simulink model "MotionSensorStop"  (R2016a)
settings: Solver=VariableStepAuto  StartTime=0.0  StopTime=10.0  RelTol=1e-3
libraries: vexarmcortexlib x3

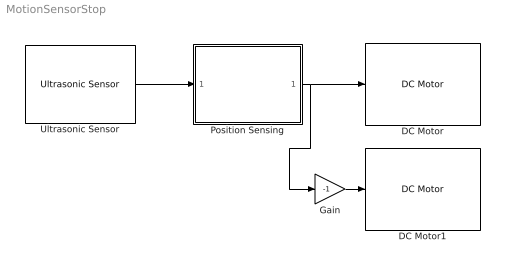
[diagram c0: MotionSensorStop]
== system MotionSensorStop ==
  DC Motor : vexarmcortexlib/DC Motor  motor=3  scaleFactor=1/13.5  SimulationOut=off
  DC Motor1 : vexarmcortexlib/DC Motor  motor=7  scaleFactor=1/13.5  SimulationOut=off
  Gain : Gain  Gain=-1
  Position Sensing : Stateflow chart  TreatAsAtomicUnit=on
  Ultrasonic Sensor : vexarmcortexlib/Ultrasonic Sensor  inputPin=3  outputPin=2  inputPortSim=off  SampleTime=0.2
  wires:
  Ultrasonic Sensor/1 -> Position Sensing/1(position)
  Position Sensing/1(speed) -> Gain/1, DC Motor/1
  Gain/1 -> DC Motor1/1

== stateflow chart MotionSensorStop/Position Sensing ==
  state Drive_Forward
    during:
    speed = 50;
  state Stop
    during:
    speed = 0;
  (default) -> Drive_Forward : {speed = 0;}
  Drive_Forward -> Stop : [position < .3 && position > 0.02]
  data: position input; speed output
